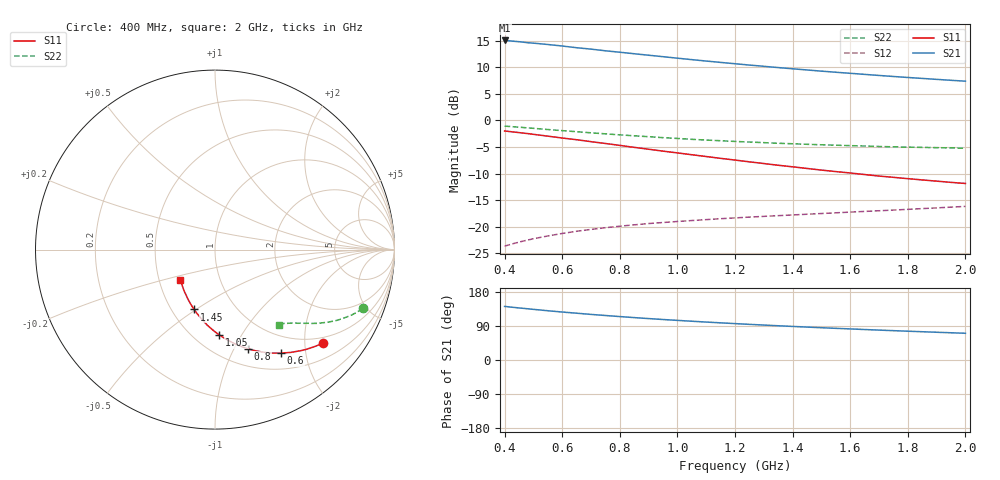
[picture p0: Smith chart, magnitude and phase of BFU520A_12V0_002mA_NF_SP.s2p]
! Filename:  P:\Prog\Test\Noise\ATS_data\Testdata_Net\06 Compressed Noise after Statistics\BFU520A_APG2013_30_A05_12p0V_002mA_NF_CM01_D.sf
! Date/Time: Wed 24/Apr/2013 20:06:20
! BFU520A_APG2013_30_A05_12p0V_1to20mA_NF_CM01_Bias2_R.sf
! Noise Parameter Data File
! BFU520A_APG2013_30_A05_12p0V_1to20mA_NF_CM01
! Date/time: Thu Apr 11 10:46:45 2013
! VAR V_out= 12.001000
! VAR I_out= 1.990000
! VAR V_in= 0.803300
! VAR I_in= 0.018700
! Device data file deembeded for feedlines and parallel
! Original file: \06 Compressed Noise after Statistics\BFU520A_APG2013_30_A05_12p0V_002mA_NF_CM01_R.sf
! Feed-files: PR017V01_150413_Feed1.s2p, PR017V01_150413_Feed2.s2p
! Parallel-file: PR017V01_150413_Par.s2p
# MHz S MA R 50
!  Freq-MHz  S11-mag  S11-arg  S21-mag  S21-arg  S12-mag  S12-arg  S22-mag  S22-arg
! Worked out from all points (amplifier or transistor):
!   37 points, 400 MHz to 2 GHz, reference 50 ohm
!   highest |S21| = 15.1 dB at 400 MHz (marker M1)
!   |S21| within 3 dB of that: start of sweep to 939.5 MHz
!   unconditionally stable (mu >= 1): nowhere
!   at 500 MHz: K = 0.35, MSG = 18.4 dB, |S12| = -22.3 dB
!   at 1.1 GHz: K = 0.69, MSG = 14.9 dB, |S12| = -18.7 dB
!   at 2 GHz: K = 0.98, MSG = 11.8 dB, |S12| = -16.2 dB
!   lowest NFmin = 0.59 dB at 433 MHz
!   S11 on the Smith chart (normalised r, x): 400 MHz: 0.86, -2.44; 600 MHz: 0.73, -1.57; 800 MHz: 0.68, -1.14; 1.05 GHz: 0.66, -0.81; 1.45 GHz: 0.64, -0.49; 2 GHz: 0.64, -0.23
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400  0.7967 -40.7  5.67 141.4  0.06549 66.7  0.8849 -21.8
420  0.7851 -42.5  5.618 139.7  0.06797 65.8  0.8768 -22.6
440  0.7743 -44.3  5.551 138.2  0.07035 65.0  0.8687 -23.4
480  0.7528 -47.6  5.399 135.2  0.07476 63.5  0.8514 -24.9
500  0.7406 -49.4  5.35 133.7  0.07696 62.8  0.8436 -25.6
550  0.7119 -53.6  5.195 130.0  0.08172 61.0  0.8217 -27.3
600  0.6835 -57.5  5.028 126.6  0.08624 59.6  0.8023 -28.8
650  0.6588 -61.1  4.843 123.5  0.09048 58.3  0.7838 -30.2
700  0.6316 -64.8  4.701 120.3  0.09417 57.2  0.7653 -31.5
750  0.6072 -68.2  4.532 117.4  0.09774 56.1  0.7484 -32.7
800  0.5826 -71.7  4.392 114.6  0.101 55.3  0.7321 -33.7
850  0.5583 -75.0  4.251 111.9  0.104 54.5  0.7171 -34.8
950  0.5143 -81.2  3.988 106.8  0.1094 53.4  0.689 -36.6
1050  0.4757 -87.2  3.74 102.3  0.1142 52.7  0.6645 -38.2
1100  0.4575 -90.1  3.629 100.1  0.1165 52.4  0.6539 -38.9
1200  0.4239 -95.7  3.423 96.0  0.1208 52.1  0.6346 -40.2
1300  0.3931 -101.1  3.238 92.2  0.125 52.0  0.6184 -41.6
1450  0.3533 -109.3  2.99 86.9  0.1309 52.3  0.5964 -43.3
1500  0.341 -112.0  2.915 85.2  0.1329 52.4  0.5903 -43.9
1650  0.3096 -119.9  2.717 80.4  0.1391 53.1  0.5747 -45.6
1750  0.2914 -125.4  2.595 77.4  0.1433 53.8  0.5647 -46.7
2000  0.2551 -138.9  2.345 70.5  0.1552 55.5  0.5483 -49.6
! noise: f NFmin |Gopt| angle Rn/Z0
400  0.6714  0.4358  17.49  0.2124
460  0.6202  0.4515  20.73  0.2144
600  0.6597  0.474  25  0.2293
800  0.6488  0.4441  37.96  0.1825
1000  0.6582  0.4565  48.45  0.1728
1200  0.7337  0.434  57.23  0.1687
1400  0.746  0.4119  68.76  0.1505
1600  0.7372  0.3817  79.12  0.13
1800  0.6657  0.361  90.74  0.1206
2000  0.7568  0.3396  107.2  0.098
